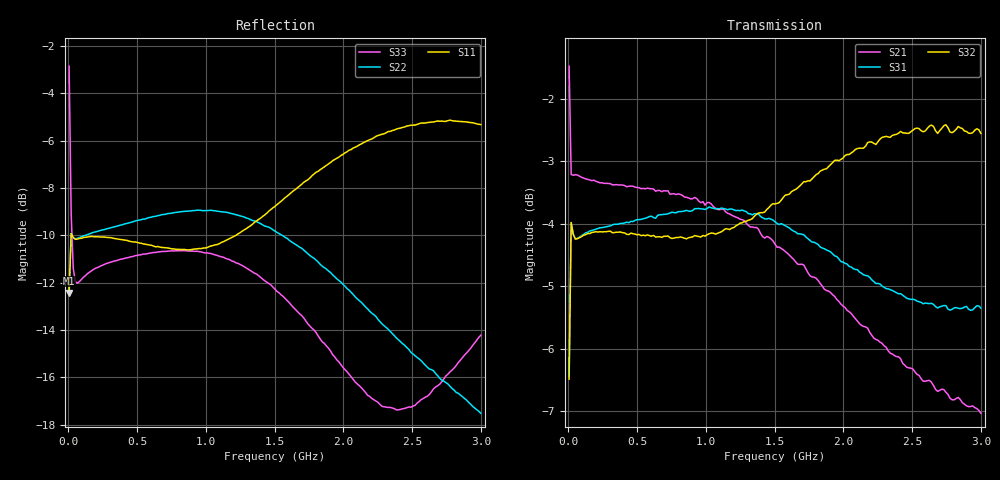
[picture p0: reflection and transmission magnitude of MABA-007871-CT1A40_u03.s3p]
#	MHz	S	RI	R	50
!FREQ	R1	I1	R2	I2	R3	I3
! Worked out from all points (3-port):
!   201 points, 5 MHz to 3 GHz, reference 50 ohm
!   strongest paths, dB at 5 MHz, 753.8 MHz, 1.502 GHz, 2.251 GHz, 3 GHz:
!     S32: -6.5, -4.2, -3.7, -2.7, -2.6
!     S31: -6.4, -3.8, -4.0, -5.0, -5.3
!     S21: -1.5, -3.5, -4.3, -5.9, -7.0
!   lowest |S11| = -12.4 dB at 5 MHz (marker M1), VSWR 1.63, Z = 66.8 + j23 ohm
!   |S11| at or under -10 dB: start of sweep to 19.51 MHz; 26.77 MHz to 1.218 GHz (1.191 GHz wide, 191 % of centre)
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5  0.1758 0.1621  0.8253 -0.1679  -0.3505 -0.3232
   0.8267 -0.1689  0.1729 0.1639  0.3488 0.3243
   -0.3505 -0.3232  0.3447 0.3257  -0.3036 0.6534
19.975  0.315 0.0512  0.6873 -0.0773  -0.6227 -0.1084
        0.6868 -0.0774  0.3133 0.0623  0.6211 0.1196
        -0.6227 -0.1084  0.6214 0.1192  0.2488 0.2472
34.95  0.3126 0.0107  0.6878 -0.0569  -0.6181 -0.0345
       0.6878 -0.0573  0.3115 0.0296  0.6165 0.053
       -0.6181 -0.0345  0.617 0.0528  0.2412 0.1208
94.85  0.3097 -0.0372  0.6824 -0.087  -0.6165 0.0347
       0.6821 -0.0872  0.3139 0.0129  0.6163 0.0158
       -0.6165 0.0347  0.6163 0.0159  0.2469 0.0648
768.725  0.0127 -0.2958  0.4323 -0.5117  -0.4219 0.4868
         0.4358 -0.505  0.3441 -0.0797  0.6095 -0.0919
         -0.4219 0.4868  0.6081 -0.0908  0.2917 -0.0293
1113.15  -0.2198 -0.2124  0.1819 -0.6237  -0.1997 0.6183
         0.1935 -0.6187  0.3202 -0.1524  0.6129 -0.1219
         -0.1997 0.6183  0.61 -0.1216  0.2749 -0.0753
1502.5  -0.3594 0.0587  -0.1276 -0.5864  0.0868 0.6275
        -0.1144 -0.5971  0.2429 -0.2126  0.6355 -0.1738
        0.0868 0.6275  0.631 -0.1745  0.2188 -0.1068
1802  -0.308 0.3003  -0.3097 -0.4593  0.2667 0.5473
      -0.3069 -0.4814  0.1719 -0.2215  0.6558 -0.2378
      0.2667 0.5473  0.6498 -0.2348  0.1711 -0.0975
2251.25  -0.0208 0.5137  -0.4435 -0.1974  0.4323 0.3644
         -0.4637 -0.2106  0.0924 -0.1887  0.6428 -0.3758
         0.4323 0.3644  0.6364 -0.3661  0.1327 -0.046
3000  0.4523 0.2991  -0.3816 0.2046  0.5369 0.0612
      -0.3833 0.2264  0.0401 -0.1269  0.4712 -0.5945
      0.5369 0.0612  0.4725 -0.5765  0.1934 0.0221
